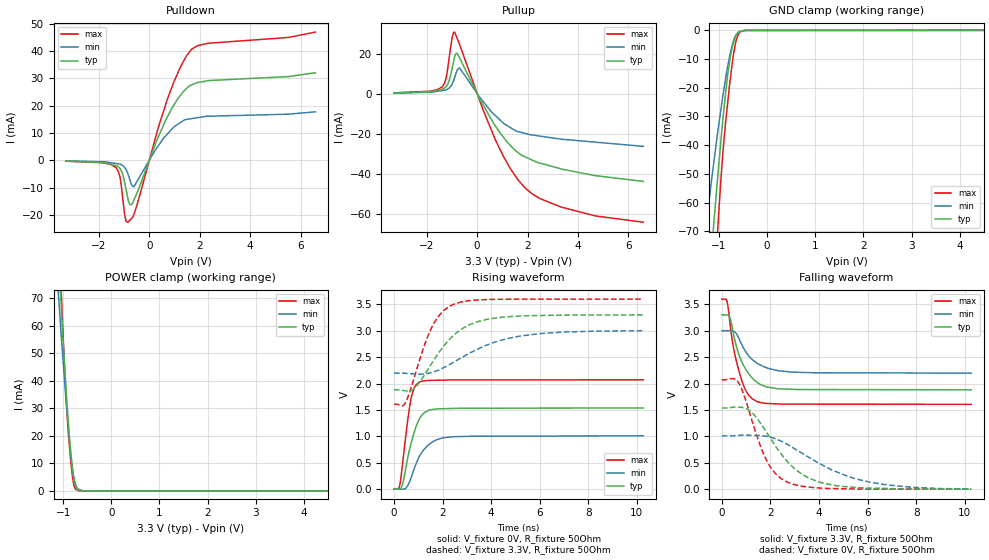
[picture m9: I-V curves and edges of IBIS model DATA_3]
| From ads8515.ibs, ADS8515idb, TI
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|   DATA OUTPUT Model  3.3V
[Model] DATA_3
Model_type 3-state
Polarity   Non-Inverting
Enable   Active-Low
Vmeas = 1.65
Vref = 1.65
Cref = 15pF
Rref = 50
|   typ   min   max
| AVERAGE
C_comp   9.7302320E-12  8.5643450E-12  1.0799656E-11
| HIGH out
|C_comp   1.0844090e-11  9.5659310e-12  1.1952090e-11
| LOW out
|C_comp   8.6163740e-12  7.5627590e-12  9.6472220e-12
[Voltage Range]   3.3   3   3.6
[Temperature Range]   27   85   -40
[Pullup Reference]   3.3   3   3.6
[Pulldown Reference]   0   0   0
[Power Clamp Reference]   3.3   3   3.6
[GND Clamp Reference]   0   0   0
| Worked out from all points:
|   slope of the pulldown table from 0 to 0.495 V, typ, clamps not added: 43.2 ohm
|   slope of the pullup table from 0 to 0.495 V, typ, clamps not added: 43.3 ohm
|   GND clamp passes 1 mA (typ) near -0.61 V on its own axis
|   POWER clamp passes 1 mA (typ) near -0.72 V on its own axis
|   falling waveform, V_fixture 3.3V, R_fixture 50Ohm: 20-80 % time 693ps typ, 841ps min, 542ps max; typ from 3.3 V to 1.88 V
|   rising waveform, V_fixture 0V, R_fixture 50Ohm: 20-80 % time 496ps typ, 656ps min, 344ps max; typ from 0 V to 1.54 V
|   rising waveform, V_fixture 3.3V, R_fixture 50Ohm: 20-80 % time 1.49ns typ, 2.3ns min, 962ps max; typ from 1.88 V to 3.3 V
|   falling waveform, V_fixture 0V, R_fixture 50Ohm: 20-80 % time 1.6ns typ, 2.63ns min, 1ns max; typ from 1.54 V to 0 V
[Pulldown]
|   Voltage   I  typ   I  min   I  max
-3.3V     -285.2uA   -205.1uA   -305.9uA
-1.332V   -1.915mA   -1.132mA   -2.548mA
-1.168V   -2.944mA   -1.363mA   -5.815mA
-1.065V   -4.683mA   -1.862mA   -12.67mA
-951.4mV  -9.087mA   -2.898mA   -20.99mA
-849.3mV  -13.75mA   -4.825mA   -22.6mA
-724.6mV  -16.23mA   -8.407mA   -21.44mA
-602.2mV  -14.4mA    -9.512mA   -19.6mA
713mV     15.77mA    9.561mA    22.16mA
1.224V    23.58mA    13.72mA    33.82mA
1.661V    27.49mA    15.22mA    40.43mA
6.59V     32.02mA    17.73mA    46.86mA
[GND Clamp]
|   Voltage   I  typ   I  min   I  max
-3.3V     -591.1mA   -422.7mA   -812mA
-1.277V   -103.1mA   -69.39mA   -145.8mA
-1.256V   -98.71mA   -66.5mA    -139.3mA
-1.13V    -71.91mA   -49.03mA   -100mA
-1.031V   -52.04mA   -36.07mA   -70.99mA
-1.008V   -47.58mA   -33.28mA   -64.39mA
-909mV    -29.48mA   -21.72mA   -40.61mA
-811.6mV  -14.52mA   -11.9mA    -23.99mA
-695mV    -4.049mA   -3.458mA   -8.04mA
-592.6mV  -692.3uA   -489.7uA   -1.321mA
-451.3mV  -25.39uA   -38.04uA   -20.87uA
6.59V     0A         0A         0A
[Pullup]
|   Voltage   I  typ   I  min   I  max
-3.3V     365.8uA    284.3uA    421.3uA
-1.382V   2.283mA    1.571mA    3.469mA
-1.228V   3.633mA    1.909mA    7.912mA
-1.121V   5.954mA    2.689mA    16.8mA
-992mV    12.62mA    4.739mA    27.87mA
-903.5mV  17.77mA    7.615mA    30.72mA
-806.4mV  20.18mA    11.29mA    28.04mA
-680.8mV  17.43mA    12.64mA    24mA
713mV     -15.93mA   -10.78mA   -22.73mA
1.877V    -31.36mA   -19.73mA   -46.68mA
3.305V    -37.41mA   -22.65mA   -56.43mA
6.59V     -43.77mA   -26.27mA   -64.08mA
[POWER Clamp]
|   Voltage   I  typ   I  min   I  max
-3.3V     1.008A     842.3mA    1.242A
-1.108V   90.57mA    73.77mA    103.7mA
-1.076V   79.59mA    65.68mA    88.94mA
-1.053V   71.4mA     59.65mA    78.53mA
-1.04V    67.23mA    56.36mA    72.8mA
-934.6mV  35.65mA    31.97mA    32.32mA
-893.3mV  25.12mA    23.24mA    21.28mA
-849.3mV  15.5mA     14.8mA     12.04mA
-803.1mV  7.427mA    7.794mA    4.759mA
-765.5mV  3.266mA    3.848mA    1.493mA
-665.8mV  340uA      538.7uA    15.4uA
6.59V     0A         0A         0A
[Ramp]
R_load = 50
|   typ   min   max
dV/dt_r   0.922229/4.9411e-010   0.60548/6.51598e-010   1.24254/3.4265e-010
dV/dt_f   0.851357/6.89426e-010  0.481832/8.27711e-010   1.19615/5.41062e-010
[Falling Waveform]
V_fixture = 3.3V
V_fixture_min = 3V
V_fixture_max = 3.6V
R_fixture = 50Ohm
C_fixture = 0F
|   Time   V  typ   V  min   V  max
0s        3.3V       3V         3.6V
219.5ps   3.3V       3.001V     3.546V
353.3ps   3.216V     3.001V     3.071V
489.9ps   2.917V     2.99V      2.656V
833.2ps   2.4V       2.722V     2.041V
1.094ns   2.196V     2.531V     1.788V
1.43ns    2.031V     2.391V     1.663V
1.847ns   1.936V     2.299V     1.623V
2.889ns   1.891V     2.217V     1.61V
10.27ns   1.881V     2.197V     1.606V
[Rising Waveform]
V_fixture = 0V
V_fixture_min = 0V
V_fixture_max = 0V
R_fixture = 50Ohm
C_fixture = 0F
|   Time   V  typ   V  min   V  max
0s        -444.3nV   -2.516uV   -2.383uV
233.1ps   -784.4uV   -1.19mV    61.86mV
358.5ps   98.19mV    -1.829mV   489.8mV
553.1ps   552.7mV    53.37mV    1.249V
694.4ps   844.4mV    200mV      1.684V
848.9ps   1.095V     402.8mV    1.925V
1.071ns   1.347V     636.6mV    2.03V
1.574ns   1.507V     890.7mV    2.06V
2.472ns   1.528V     992.2mV    2.067V
10.27ns   1.537V     1.009V     2.071V
[Rising Waveform]
V_fixture = 3.3V
V_fixture_min = 3V
V_fixture_max = 3.6V
R_fixture = 50Ohm
C_fixture = 0F
|   Time   V  typ   V  min   V  max
0s        1.881V     2.197V     1.606V
461.9ps   1.863V     2.194V     1.626V
821.7ps   1.901V     2.181V     2.091V
1.234ns   2.146V     2.181V     2.699V
1.546ns   2.372V     2.206V     3.053V
1.952ns   2.651V     2.279V     3.337V
2.455ns   2.911V     2.404V     3.5V
3.508ns   3.18V      2.664V     3.584V
5.17ns    3.278V     2.897V     3.598V
10.27ns   3.3V       3V         3.6V
[Falling Waveform]
|Gnd
V_fixture = 0V
V_fixture_min = 0V
V_fixture_max = 0V
R_fixture = 50Ohm
C_fixture = 0F
|   Time   V  typ   V  min   V  max
0s        1.537V     1.009V     2.071V
685.4ps   1.552V     1.018V     2.022V
1.155ns   1.487V     1.02V      1.428V
1.82ns    1.09V      1.003V     564.7mV
2.211ns   814.7mV    953.9mV    291.2mV
2.701ns   521.8mV    848.5mV    132.3mV
3.94ns    144.1mV    504.8mV    24.77mV
5.623ns   29.41mV    182.6mV    3.888mV
7.691ns   5.126mV    40.61mV    1.161mV
10.27ns   -444.3nV   -2.516uV   -2.383uV
